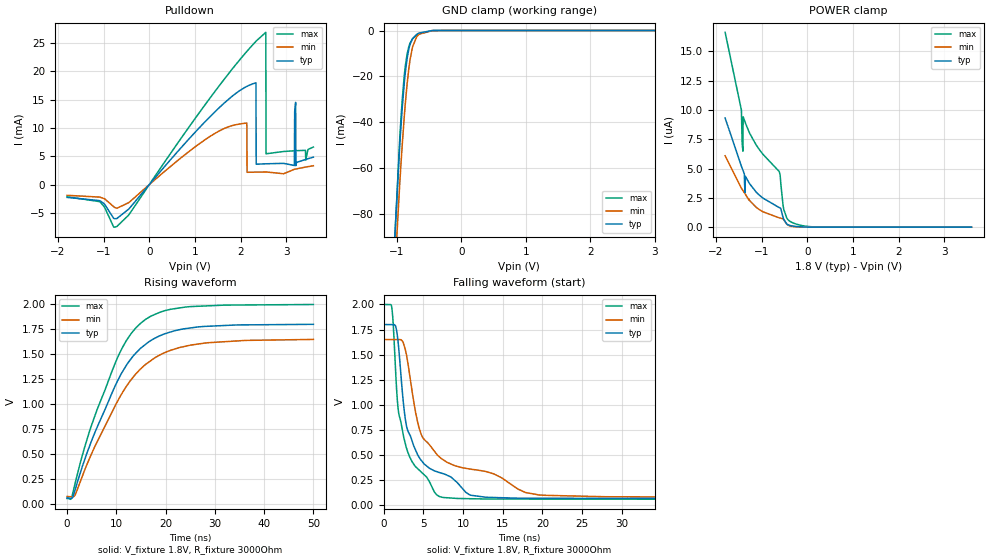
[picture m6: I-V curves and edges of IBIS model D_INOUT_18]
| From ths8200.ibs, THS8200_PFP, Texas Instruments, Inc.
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[Model]   D_INOUT_18
Model_type   I/O_open_drain
Polarity   Non-Inverting
Enable   Active-Low
Vinl = .4
Vinh = .95
Vmeas = 1.0
Vref = 0
Cref = 0pF
Rref = 3000
|   typ   min   max
|   (nom PVT)   (Fast PVT)   (slow PVT)
C_comp   1.235p   0.985p   1.478p
|C_comp (ON state)   1.385p   1.101p   1.606p
|C_comp (OFF state)   1.235p   0.985p   1.478p
| Where   nom PVT is  Nominal Process, 1.8V, 27C
|   Fast PVT is Strong Process, 2.0V, 0C
|   Slow PVT is Weak Process, 1.65V, 85C
[Voltage Range]   1.8   1.65   2
[Temperature Range]   27   85   0
[Pullup Reference]   1.8   1.65   2
[Pulldown Reference]   -0   -0   -0
[Power Clamp Reference]   1.8   1.65   2
[GND Clamp Reference]   -0   -0   -0
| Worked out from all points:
|   slope of the pulldown table from 0 to 0.27 V, typ, clamps not added: 105 ohm
|   GND clamp passes 1 mA (typ) near -0.64 V on its own axis
|   falling waveform, V_fixture 1.8V, R_fixture 3000Ohm: 20-80 % time 3.08ns typ, 5.76ns min, 2.16ns max; typ from 1.8 V to 0.06 V
|   rising waveform, V_fixture 1.8V, R_fixture 3000Ohm: 20-80 % time 9.62ns typ, 10.6ns min, 8.87ns max; typ from 0.06 V to 1.8 V
[Pulldown]
|   Voltage   I(typ)   I(min)   I(max)
-1.8V     -2.248mA   -1.884mA   -2.135mA
-709.2mV  -5.971mA   -4.165mA   -7.374mA
1.818V    15.59mA    10.4mA     20.38mA
2.336V    17.94mA    2.203mA    25.25mA
2.342V    3.599mA    2.204mA    25.3mA
2.552V    3.673mA    2.226mA    26.84mA
2.558V    3.674mA    2.227mA    5.433mA
3.179V    3.376mA    2.7mA      5.965mA
3.184V    12.78mA    2.709mA    5.968mA
3.206V    14.5mA     2.746mA    5.976mA
3.211V    3.337mA    2.755mA    5.978mA
3.595V    4.844mA    3.33mA     6.633mA
[GND Clamp]
|   Voltage   I(typ)   I(min)   I(max)
-1.8V     -597mA     -576.1mA   -647.7mA
-1.055V   -103.3mA   -118.2mA   -104.7mA
-952.2mV  -49.72mA   -66.46mA   -46.76mA
-914.4mV  -33.79mA   -49.87mA   -30.29mA
-882mV    -22.67mA   -37.24mA   -19.46mA
-865.8mV  -18.14mA   -31.59mA   -15.32mA
-838.8mV  -12.18mA   -23.29mA   -10.22mA
-790.2mV  -5.855mA   -12.27mA   -5.336mA
-752.4mV  -3.498mA   -7.019mA   -3.567mA
-687.6mV  -1.625mA   -2.653mA   -1.94mA
-428.4mV  -13.3uA    -27.78uA   -18.32uA
3.595V    0A         0A         0A
[POWER Clamp]
|   Voltage   I(typ)   I(min)   I(max)
-1.8V     9.317uA    6.092uA    16.63uA
-1.444V   5.198uA    3.329uA    9.996uA
-1.427V   5.041uA    3.228uA    7.153uA
-1.411V   4.873uA    3.128uA    6.483uA
-1.406V   4.816uA    3.095uA    9.421uA
-1.379V   4.533uA    2.934uA    9.137uA
-1.363V   2.942uA    2.84uA     8.965uA
-1.357V   4.343uA    2.809uA    8.908uA
-617.4mV  1.674uA    796.5nA    4.758uA
-514.8mV  644.5nA    638.2nA    1.505uA
-396mV    162.4nA    123.9nA    541.9nA
3.595V    0A         0A         0A
[Ramp]
R_load = 3000
|   typ   min   max
dV/dt_r   1.04219/9.60085e-09   0.943053/1.05639e-08   1.16492/8.86798e-09
dV/dt_f   1.04387/3.08109e-09   0.945094/5.75318e-09   1.16751/2.16109e-09
[Falling Waveform]
V_fixture = 1.8V
V_fixture_min = 1.65V
V_fixture_max = 2V
R_fixture = 3000Ohm
C_fixture = 0F
|   Time   V(typ)   V(min)   V(max)
0s        1.8V       1.65V      2V
995.8ps   1.799V     1.65V      1.977V
1.546ns   1.767V     1.65V      1.248V
1.869ns   1.573V     1.65V      919.4mV
2.806ns   810.8mV    1.515V     580.2mV
4.425ns   477.9mV    773.3mV    348.7mV
6.997ns   321.5mV    479.1mV    82.15mV
11.01ns   94.01mV    354.6mV    59.92mV
19.55ns   64.66mV    97.86mV    56.44mV
50ns      60.17mV    74.8mV     53.92mV
[Rising Waveform]
V_fixture = 1.8V
V_fixture_min = 1.65V
V_fixture_max = 2V
R_fixture = 3000Ohm
C_fixture = 0F
|   Time   V(typ)   V(min)   V(max)
0s        60.05mV    74.16mV    53.94mV
835.3ps   54.58mV    71.61mV    50.95mV
1.632ns   141.5mV    90.24mV    206.1mV
4.814ns   611.1mV    484.8mV    766.4mV
9.985ns   1.205V     1.004V     1.435V
12.01ns   1.385V     1.174V     1.633V
15.01ns   1.561V     1.355V     1.811V
19.55ns   1.697V     1.508V     1.929V
25.11ns   1.761V     1.589V     1.975V
50ns      1.797V     1.646V     1.995V
